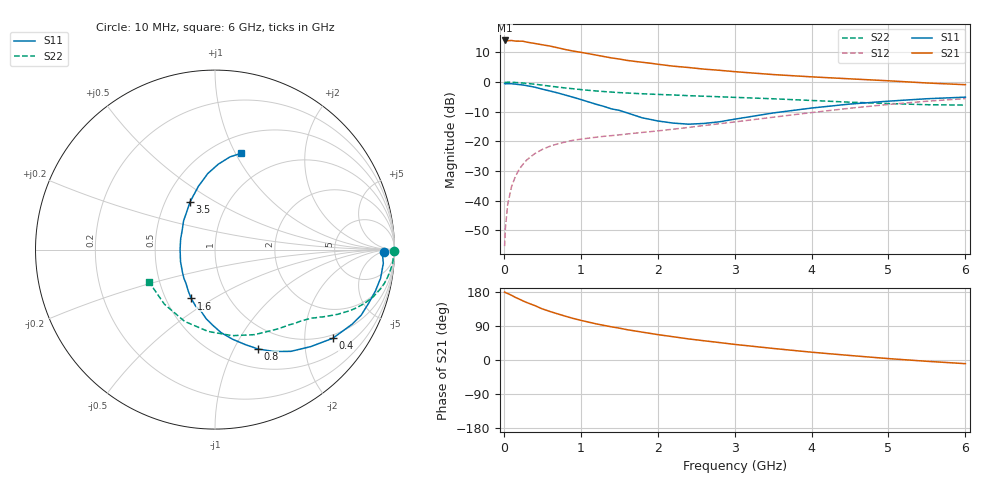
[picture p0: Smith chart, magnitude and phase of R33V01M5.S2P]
! SIEMENS Small Signal Semiconductors
! BFR181
! Si NPN RF Bipolar Junction Transistor in SOT23
! VCE = 3 V  IC = 1.5 mA
! Common Emitter S-Parameters:  May  1996
# GHz  S  MA  R  50
!  f  S11  S21  S12  S22
! GHz  MAG  ANG  MAG  ANG  MAG  ANG  MAG  ANG
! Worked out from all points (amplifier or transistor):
!   36 points, 10 MHz to 6 GHz, reference 50 ohm
!   highest |S21| = 14.0 dB at 10 MHz (marker M1)
!   |S21| within 3 dB of that: start of sweep to 789.5 MHz
!   unconditionally stable (mu >= 1): 1.759 GHz to 3.526 GHz
!   at 250 MHz: K = 0.19, MSG = 20.7 dB, |S12| = -27.7 dB
!   at 1.4 GHz: K = 0.89, MSG = 13.1 dB, |S12| = -18.1 dB
!   at 6 GHz: K = 0.86, MSG = 2.3 dB, |S12| = -5.6 dB
!   S11 on the Smith chart (normalised r, x): 10 MHz: 31, -8; 400 MHz: 0.90, -2.73; 800 MHz: 0.72, -1.25; 1.6 GHz: 0.67, -0.40; 3.5 GHz: 0.67, +0.39; 6 GHz: 0.68, +1.06
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0.01  0.9423 -0.9  5.039 179.3  0.0017 89.1  0.9984 -0.5
0.02  0.9341 -1.8  4.938 178.0  0.0034 87.4  0.9884 -1.0
0.05  0.9409 -4.7  4.986 175.4  0.0086 88.5  0.9952 -2.3
0.1  0.9363 -9.8  5.033 170.8  0.0172 83.7  0.9924 -4.5
0.15  0.9229 -14.5  4.913 165.2  0.0255 80.5  0.9833 -6.8
0.25  0.8925 -24.2  4.887 155.9  0.0412 75.2  0.9634 -11.1
0.3  0.8694 -28.6  4.717 151.5  0.0488 72.5  0.9498 -13.1
0.4  0.8213 -37.0  4.493 143.8  0.0617 67.4  0.921 -16.5
0.5  0.7592 -45.4  4.258 134.9  0.0731 63.6  0.8874 -19.6
0.6  0.7071 -53.3  4.052 128.0  0.0827 60.2  0.8536 -22.3
0.8  0.6033 -66.6  3.542 115.6  0.0975 54.6  0.7943 -26.3
0.9  0.5549 -72.4  3.34 109.8  0.1042 53.1  0.7713 -27.9
1.1  0.463 -85.9  3.017 100.0  0.1131 50.7  0.726 -30.7
1.3  0.3888 -97.2  2.7 91.4  0.1214 49.7  0.6917 -32.9
1.6  0.303 -116.0  2.323 80.1  0.1328 49.4  0.6547 -36.0
1.9  0.235 -137.7  2.084 70.3  0.1454 50.6  0.6266 -39.3
2.2  0.2032 -161.0  1.856 61.4  0.1601 51.8  0.6055 -42.8
2.8  0.2134 148.7  1.582 46.1  0.1981 53.6  0.5652 -51.2
3.5  0.3009 117.4  1.339 30.5  0.2551 52.7  0.5225 -65.1
4.5  0.4258 95.4  1.134 11.9  0.3619 45.8  0.4578 -94.7
5.5  0.5234 80.8  0.965 -3.4  0.4747 33.4  0.4147 -132.9
6  0.5565 74.7  0.903 -9.7  0.5261 25.8  0.4088 -153.4
